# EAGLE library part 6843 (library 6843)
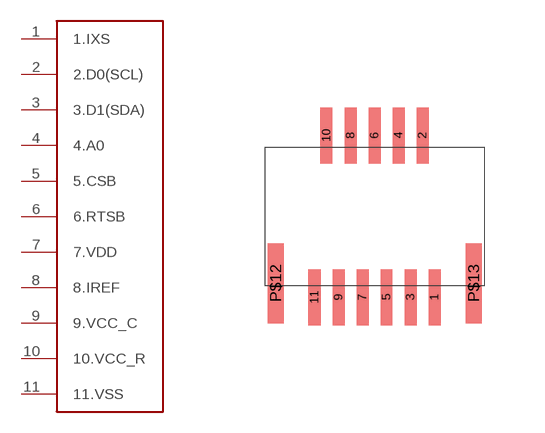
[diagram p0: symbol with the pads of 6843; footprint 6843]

Designator prefix -

## 6843  [6843]
1  1.IXS
2  2.D0(SCL)
3  3.D1(SDA)
4  4.A0
5  5.CSB
6  6.RTSB
7  7.VDD
8  8.IREF
9  9.VCC_C
10  10.VCC_R
11  11.VSS

## Footprint 6843 (pad centres in mm)
smd 0.3 x 1.4: 1 -1.25,-3.75; 2 -1.55,0.3; 3 -1.85,-3.75; 4 -2.15,0.3; 5 -2.45,-3.75; 6 -2.75,0.3; 7 -3.05,-3.75; 8 -3.35,0.3; 9 -3.65,-3.75; 10 -3.95,0.3; 11 -4.25,-3.75
smd 0.4 x 2: P$12 -5.22,-3.4; P$13 -0.27,-3.4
